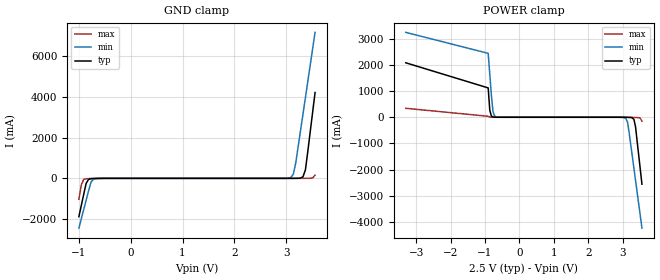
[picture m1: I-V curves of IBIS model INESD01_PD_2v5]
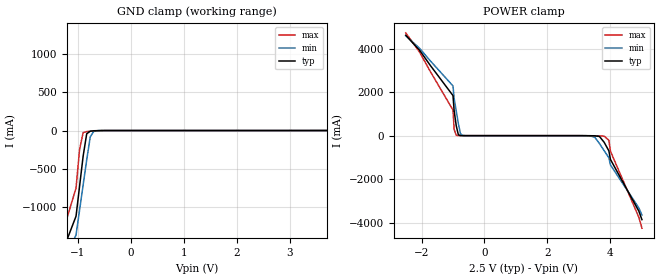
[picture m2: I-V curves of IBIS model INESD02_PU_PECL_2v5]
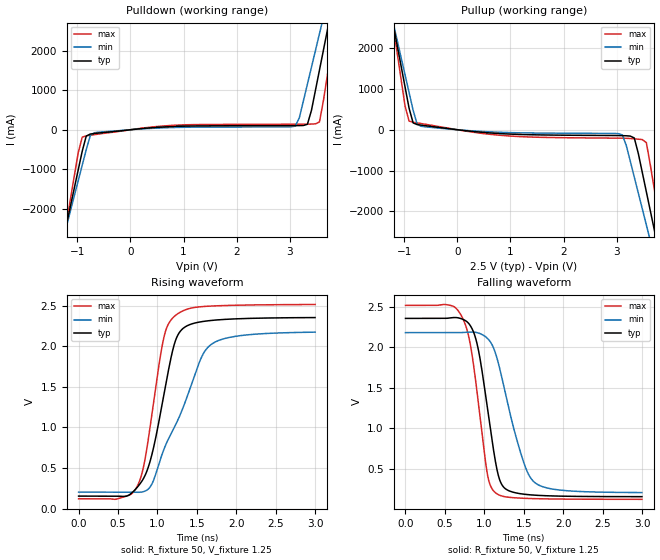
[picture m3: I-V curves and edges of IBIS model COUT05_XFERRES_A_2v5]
|   This file is an IBIS representation of the   |
|   Integrated Device Technology , Inc.   |
|   ICS87946I-147   |
|   LOW SKEW, Div1, Div2 LVCMOS/LVTTL CLOCK GENERATOR   |
[IBIS Ver]   4.1
[File name]   87946i_147.ibs
[File Rev]   1.0
[Date]   22 Jun 2009 | Last modified
|   May 23 2003 | Generated
[Source]   Originated at Integrated Device Technology, Inc.
[Disclaimer]
IDT hereby grants the user of this IBIS model a non-exclusive,
nontransferable license to use this IBIS model under the following terms.
Before using this IBIS model, the user should read this license.
If the user does not accept these terms,  the IBIS model should be
returned to IDT within 30 days.
   The user is granted this license only to use the IBIS model and
is not granted rights to sell, load, rent, lease or license the IBIS
model in whole or in part, or in modified form to anyone other than
user. User may modify the IBIS model to suit its specific
applications but rights to derivative works and such modifications
shall belong to IDT.
   This IBIS model is provided on an "AS IS" basis and IDT makes
absolutely no warranty with respect to the information contained
herein. IDT DISCLAIMS AND CUSTOMER WAIVES ALL WARRANTIES, EXPRESS
OR IMPLIED, INCLUDING WARRANTIES OF MERCHANTABILITY OR FITNESS FOR
A PARTICULAR PURPOSE. The entire risk as to quality and performance
is with the Customer. ACCORDINGLY, IN NO EVENT SHALL THE COMPANY BE
LIABLE FOR ANY DAMAGES, WHETHER IN CONTRACT OR TORT,INCLUDING ANY
LOST PROFITS OR OTHER INCIDENTAL, CONSEQUENTIAL, EXEMPLARY, OR
PUNITIVE DAMAGES ARISING OUT OF THE USE OR APPLICATION OF THE IBIS
model provided in this package. Further, IDT reserves the right to
make changes without notice to any product herein to improve
reliability, function, or design. IDT does not convey any license
under patent rights or any other intellectual property rights,
including those of third parties.
   IDT is not obligated to provide maintenance or support
for the licensed IBIS model.
[Copyright]   Copyright 2004 by Integrated Device Technology , Inc.
[Component]   ICS87946I-147
[Manufacturer] Integrated Device Technology, Inc.
[Package]
|LQFP32
|lead+wire   typ   min   max
R_pkg   220.4m   212.5m   238m
L_pkg   1.841n   1.708n   1.974n
C_pkg   0.316p   0.2907p   0.33p
[Pin]   signal_name   model_name   R_pin   L_pin   C_pin
1   CLK_SEL   INESD01_PD   238m   1.974n   0.330p
2   VDD   POWER   225m   1.841n   0.311p
3   CLK0   INESD02_PU_PECL   218m   1.7745n   0.301p
4   CLK1   INESD02_PU_PECL   213m   1.708n   0.291p
5   DIV_SELA   INESD01_PD   213m   1.708n   0.291p
6   DIV_SELB   INESD01_PD   218m   1.7745n   0.301p
7   DIV_SELC   INESD01_PD   225m   1.841n   0.311p
8   GND   GND   238m   1.974n   0.330p
9   VDDC   POWER   238m   1.974n   0.330p
10   QC0   COUT05_XFERRES_A   225m   1.841n   0.311p
11   GND   GND   218m   1.7745n   0.301p
12   QC1   COUT05_XFERRES_A   213m   1.708n   0.291p
13   VDDC   POWER   213m   1.708n   0.291p
14   QC2   COUT05_XFERRES_A   218m   1.7745n   0.301p
15   GND   GND   225m   1.841n   0.311p
16   QC3   COUT05_XFERRES_A   238m   1.974n   0.330p
17   VDDC   POWER   238m   1.974n   0.330p
18   VDDB   POWER   225m   1.841n   0.311p
19   QB2   COUT05_XFERRES_A   218m   1.7745n   0.301p
20   GND   GND   213m   1.708n   0.291p
21   QB1   COUT05_XFERRES_A   213m   1.708n   0.291p
22   VDDB   POWER   218m   1.7745n   0.301p
23   QB0   COUT05_XFERRES_A   225m   1.841n   0.311p
24   GND   GND   238m   1.974n   0.330p
25   VDDA   POWER   238m   1.974n   0.330p
26   QA2   COUT05_XFERRES_A   225m   1.841n   0.311p
27   GND   GND   218m   1.7745n   0.301p
28   QA1   COUT05_XFERRES_A   213m   1.708n   0.291p
29   VDDA   POWER   213m   1.708n   0.291p
30   QA0   COUT05_XFERRES_A   218m   1.7745n   0.301p
31   GND   GND   225m   1.841n   0.311p
32   MR/nOE   INESD01_PD   238m   1.974n   0.330p
[Model Selector] INESD01_PD
INESD01_PD_2v5  Buffer selection for 2v5
INESD01_PD_3v3  Buffer selection for 3v3
[Model Selector] INESD02_PU_PECL
INESD02_PU_PECL_2v5  Buffer selection for 2v5
INESD02_PU_PECL_3v3  Buffer selection for 3v3
[Model Selector] COUT05_XFERRES_A
COUT05_XFERRES_A_2v5  Buffer selection for 2v5
COUT05_XFERRES_A_3v3  Buffer selection for 3v3
| Models and submodels in the file (6): INESD01_PD_2v5 (Input), INESD02_PU_PECL_2v5 (Input), COUT05_XFERRES_A_2v5 (Output), INESD01_PD_3v3 (Input), INESD02_PU_PECL_3v3 (Input), COUT05_XFERRES_A_3v3 (Output)
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[Model] INESD01_PD_2v5
Model_type   Input
Polarity   Non-Inverting
Vinl = 0.8V
Vinh = 2.0V
|   typ   min   max
C_comp   2pF   1.5pF   2.5pF
|   typ   min   max
[Voltage range]  2.5V   2.375V   2.625V
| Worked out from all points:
|   GND clamp passes 1 mA (typ) near -0.55 V on its own axis
|   POWER clamp passes 1 mA (typ) near -0.68 V on its own axis
[GND_clamp]
|Voltage I(typ)   I(min)   I(max)
-1V       -1.886A    -2.451A    -1.028A
-953.5mV  -1.338A    -1.994A    -328mA
-907mV    -789.6mA   -1.537A    -53.04mA
-860.5mV  -251.4mA   -1.081A    -21.51mA
-767.5mV  -17.28mA   -198.8mA   -10.01mA
-674.5mV  -5.28mA    -15.38mA   -3.684mA
3.092V    224.5uA    49.06mA    51.52uA
3.139V    500.8uA    208.3mA    52.98uA
3.185V    1.252mA    774.6mA    56.66uA
3.325V    81.55mA    3.177A     200uA
3.371V    416.9mA    3.978A     464.6uA
3.557V    4.225A     7.185A     159.2mA
[POWER_clamp]
|Voltage   I(typ)   I(min)   I(max)
-3.3V     2.083A     3.246A     343.1mA
-907mV    1.122A     2.445A     37.78mA
-860.5mV  267.5mA    1.644A     5.973mA
-814mV    47.03mA    844mA      1.727mA
-767.5mV  9.66mA     215.3mA    677uA
-674.5mV  960.6uA    12.66mA    131.4uA
3.092V    -1.849mA   -49.09mA   -51.51uA
3.139V    -3.491mA   -186mA     -159.7uA
3.325V    -84.03mA   -1.955A    -5.102mA
3.371V    -365.4mA   -2.411A    -8.31mA
3.51V     -2.01A     -3.782A    -35.44mA
3.557V    -2.558A    -4.239A    -152.3mA
[Model] INESD02_PU_PECL_2v5
Model_type   Input
Polarity   Non-Inverting
Vinl = .8V
Vinh =  2V
|   typ   min   max
C_comp   2pF   1.5pF   2.5pF
|   typ   min   max
[Voltage range]  2.5V   2.375V   2.625V
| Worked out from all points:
|   GND clamp passes 1 mA (typ) near -0.59 V on its own axis
|   POWER clamp passes 1 mA (typ) near -0.70 V on its own axis
[GND_clamp]
|Voltage   I(typ)   I(min)   I(max)
-2.5V     -3.894A    -3.674A    -4.294A
-1.25V    -1.521A    -1.7A      -1.261A
-1.031V   -1.125A    -1.372A    -755.3mA
-896.9mV  -335.4mA   -714.7mA   -27.06mA
-695.9mV  -3.401mA   -10.7mA    -6.467mA
3.995V    711.6uA    10.32mA    481.3uA
4.062V    4.029mA    88.04mA    1.401mA
4.129V    40.44mA    547.3mA    3.341mA
4.196V    445.8mA    1.124A     14.79mA
4.263V    1.139A     1.7A       275.9mA
4.5V      1.832A     2.277A     1.163A
5V        3.219A     3.431A     2.937A
[POWER_clamp]
|Voltage   I(typ)   I(min)   I(max)
-2.5V     4.617A     4.594A     4.726A
-1V       1.842A     2.286A     1.176A
-963.9mV  1.149A     1.709A     289.6mA
-896.9mV  456.4mA    1.132A     15.33mA
-829.9mV  42.02mA    556.1mA    3.389mA
-762.9mV  4.159mA    91.01mA    1.421mA
-695.9mV  727.9uA    10.67mA    490.4uA
3.35V     -3.204mA   -9.193mA   -6.2mA
3.8V      -305mA     -689.5mA   -24.7mA
3.95V     -699.9mA   -1.018A    -211mA
4V        -1.095A    -1.346A    -716.4mA
5V        -3.863A    -3.649A    -4.255A
[Model] COUT05_XFERRES_A_2v5
Model_type  Output
Polarity   Non-Inverting
Vmeas = 1.25
Rref = 50
Cref = 0
Vref = 1.25
|Variable  typ   min   max
C_comp   2p   1.5p   2.5p
[Voltage Range]   2.5   2.375   2.625
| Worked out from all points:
|   slope of the pulldown table from 0 to 0.375 V, typ, clamps not added: 7.84 ohm
|   slope of the pullup table from 0 to 0.375 V, typ, clamps not added: 7.17 ohm
|   rising waveform, R_fixture 50, V_fixture 1.25: 20-80 % time 274ps typ, 488ps min, 225ps max; typ from 0.154 V to 2.35 V
|   falling waveform, R_fixture 50, V_fixture 1.25: 20-80 % time 205ps typ, 309ps min, 191ps max; typ from 2.35 V to 0.154 V
| Open source, no load
|  Voltage   I(typ)   I(min)   I(max)
[Pullup]
-2.5V     11.44A     9.986A     13.84A
-1.212V   2.607A     2.64A      2.573A
-909.1mV  526mA      911.1mA    212mA
-833.3mV  167.1mA    478.9mA    184.4mA
-681.8mV  112.7mA    84.76mA    151.8mA
3.106V    -144.5mA   -124.8mA   -207.2mA
3.333V    -201.9mA   -1.16A     -222.3mA
3.485V    -1.051A    -1.943A    -242.2mA
3.561V    -1.521A    -2.334A    -315mA
3.712V    -2.464A    -3.118A    -1.472A
3.864V    -3.407A    -3.903A    -2.677A
5V        -10.49A    -9.798A    -11.71A
[Pulldown]
-2.5V     -10.49A    -9.183A    -12.66A
-1.288V   -2.917A    -2.872A    -3.01A
-1.212V   -2.443A    -2.477A    -2.405A
-909.1mV  -543.8mA   -898.7mA   -186.9mA
-833.3mV  -160.7mA   -504.4mA   -155.1mA
-757.6mV  -109mA     -149.4mA   -139.6mA
3.106V    103.9mA    93.06mA    139.6mA
3.333V    137.9mA    1.155A     141.5mA
3.561V    1.512A     2.434A     197.9mA
3.712V    2.539A     3.288A     1.405A
3.864V    3.567A     4.143A     2.72A
5V        11.31A     10.58A     12.63A
[Ramp]
|   typ   min   max
dV/dt_r   1.762/0.433n   1.577/0.660n   1.919/0.360n
dV/dt_f   1.769/0.311n   1.585/0.457n   1.923/0.297n
R_load =   50.0000
[Rising Waveform]
R_fixture = 50
V_fixture = 1.25   | VCC_typ
V_fixture_max = 1.3125   | VCC_max
V_fixture_min = 1.1875   | VCC_min
C_fixture = 0.0p
| Time   typ   min   max
0s        154.1mV    203.2mV    121.3mV
477.4ps   154.3mV    203.2mV    116.6mV
740.9ps   259.7mV    200.8mV    269.6mV
821.5ps   368.8mV    208.9mV    507.2mV
905.2ps   578.3mV    264.4mV    996.6mV
1.079ns   1.39V      722.9mV    2.098V
1.228ns   2.067V     1.027V     2.379V
1.553ns   2.301V     1.854V     2.487V
1.693ns   2.318V     2.03V      2.495V
2.998ns   2.352V     2.173V     2.513V
[Falling Waveform]
R_fixture = 50
V_fixture = 1.25   | VCC_typ
V_fixture_max = 1.3125   | VCC_max
V_fixture_min = 1.1875   | VCC_min
C_fixture = 0.0p
| Time   typ   min   max
0s        2.355V     2.179V     2.515V
725.4ps   2.344V     2.181V     2.356V
818.4ps   2.271V     2.187V     2.053V
911.4ps   2.026V     2.178V     1.415V
1.039ns   1.249V     2.109V     432mV
1.141ns   587mV      1.926V     202.8mV
1.259ns   258.4mV    1.464V     154.1mV
1.479ns   187.7mV    638mV      135.2mV
1.624ns   173.7mV    341.8mV    130.1mV
2.998ns   154.5mV    205mV      121.5mV
